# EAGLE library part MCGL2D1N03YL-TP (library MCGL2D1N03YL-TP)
N-Channel MOSFET Source: Datasheet
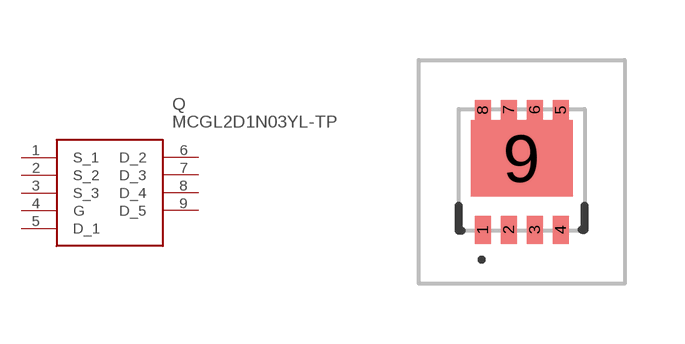
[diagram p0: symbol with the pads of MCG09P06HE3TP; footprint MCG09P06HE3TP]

Designator prefix Q

## MCGL2D1N03YL-TP (Description: N-Channel MOSFET; Height: 0.85mm; Manufacturer_Name: MCC; Manufacturer_Part_Number: MCGL2D1N03YL-TP)  [MCG09P06HE3TP]
1  S_1
2  S_2
3  S_3
4  G
5  D_1
6  D_2
7  D_3
8  D_4
9  D_5

## Footprint MCG09P06HE3TP (pad centres in mm)
PDFN3333-B
smd 0.4 x 0.7: 1 -0.975,-1.5; 2 -0.325,-1.5; 3 0.325,-1.5; 4 0.975,-1.5
smd 0.4 x 0.5: 5 0.975,1.5; 6 0.325,1.5; 7 -0.325,1.5; 8 -0.975,1.5
smd 2.55 x 1.92: 9 0,0.29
